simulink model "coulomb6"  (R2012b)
settings: Solver=ode2  StartTime=0.0  StopTime=100  FixedStep=0.001  MaxStep=0.001  RelTol=1e-3
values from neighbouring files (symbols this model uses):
  c = 2200    [coulomb_1.m]    (also in coulomb_10.m = 0.1; coulomb_11.m = 0; coulomb_2.m; coulomb_3.m)
  FG = 500    [coulomb_1.m]    (also in coulomb_10.m = 10; coulomb_11.m = 10; coulomb_2.m; coulomb_3.m)
  k = 10    [coulomb_10.m]    (also in coulomb_11.m; diff_filter_1.m = 250; diff_filter_2.m = 250; dry_friction_1.m = 2200)
  m = 400    [coulomb_1.m]    (also in coulomb_10.m = 10; coulomb_11.m = 10; coulomb_2.m; coulomb_3.m)

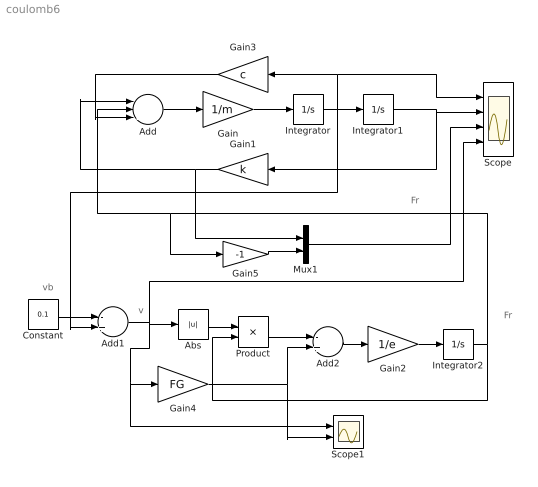
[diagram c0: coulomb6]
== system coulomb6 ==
  note: v
  note: vb
  note: Fr
  note: Fr
  Abs : Abs
  Add : Sum  Inputs=---
  Add1 : Sum  Inputs=-+
  Add2 : Sum  Inputs=-+
  Constant : Constant  Value=0.1
  Gain : Gain  Gain=1/m
  Gain1 : Gain  Gain=k
  Gain2 : Gain  Gain=1/e
  Gain3 : Gain  Gain=c
  Gain4 : Gain  Gain=FG
  Gain5 : Gain  Gain=-1
  Integrator : Integrator
  Integrator1 : Integrator
  Integrator2 : Integrator
  Mux1 : Mux  Inputs=2
  Product : Product
  Scope : Scope  NumInputPorts=4
  Scope1 : Scope  NumInputPorts=2
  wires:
  Add/1 -> Gain/1
  Gain/1 -> Integrator/1
  Integrator1/1 -> Gain1/1, Scope/2
  Constant/1 -> Add1/1
  Integrator/1 -> Add1/2, Integrator1/1, Scope/1, Gain3/1
  Gain3/1 -> Add/3
  Integrator2/1 -> Product/2, Gain5/1, Add/2
  Gain1/1 -> Mux1/1, Add/1
  Mux1/1 -> Scope/3
  Gain2/1 -> Integrator2/1
  Abs/1 -> Product/1
  Product/1 -> Add2/1
  Add2/1 -> Gain2/1
  Add1/1 -> Scope1/1, Gain4/1, Abs/1, Scope/4
  Gain4/1 -> Scope1/2, Add2/2
  Gain5/1 -> Mux1/2
